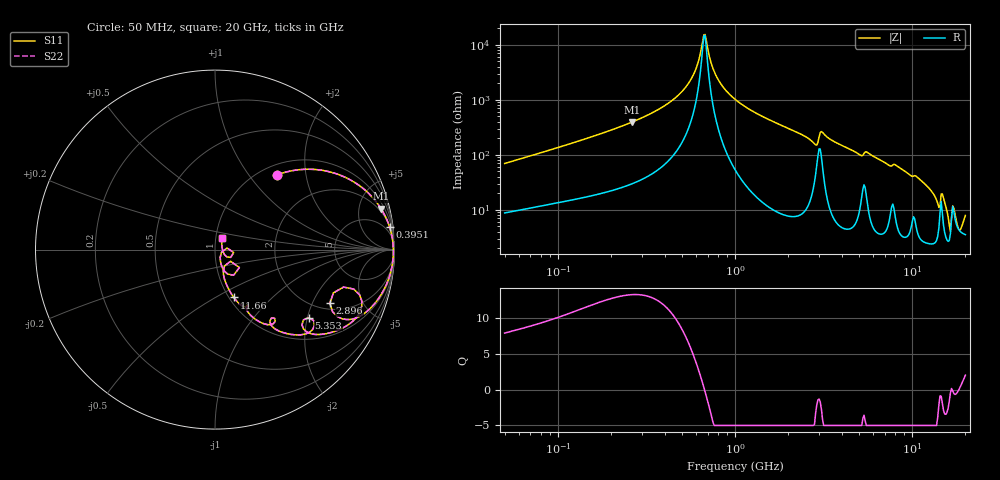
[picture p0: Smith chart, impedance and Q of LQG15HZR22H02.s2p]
!Murata Part Number: LQG15HZR22H02
!These Parameters are Measured in Series Mode Connection
!  o--[Z]--o
!Port1  Port2
!  o-------o
!Freq. Start=50[MHz] Stop=20[GHz], 401[Steps]
# Hz S RI R 50
!Freq.(Hz) S11(Real) S11(Imag) S21(Real) S21(Imag) S12(Real) S12(Imag) S22(Real) S22(Imag)
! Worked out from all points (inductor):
!   401 points, 50 MHz to 20 GHz, reference 50 ohm
!   read as one part in series: L = 215 nH near 51.52 MHz
!   highest Q = 13.2 at 263.7 MHz (marker M1), where L = 240 nH
!   self-resonance near 667.4 MHz
!   S11 on the Smith chart (normalised r, x): 50 MHz: 1.18, +1.38; 395.1 MHz: 2, +15; 2.896 GHz: 2.29, -2.73; 5.353 GHz: 1.57, -2.04; 11.66 GHz: 1.05, -0.61; 20 GHz: 1.07, +0.14
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5e7  0.3448 0.416  0.6552 -0.416  0.6552 -0.416  0.3448 0.416
1.364002e8  0.757 0.3868  0.243 -0.3868  0.243 -0.3868  0.757 0.3868
2.636584e8  0.9254 0.2276  0.0746 -0.2276  0.0746 -0.2276  0.9254 0.2276
3.721004e8  0.9678 0.1405  0.0322 -0.1405  0.0322 -0.1405  0.9678 0.1405
3.95076e8  0.9728 0.1258  0.0272 -0.1258  0.0272 -0.1258  0.9728 0.1258
5.575697e8  0.9907 0.0438  0.00933 -0.0438  0.00933 -0.0438  0.9907 0.0438
6.774326e8  0.9938 -0.00171  0.00619 0.00171  0.00619 0.00171  0.9938 -0.00171
7.868965e8  0.993 -0.037  0.00696 0.037  0.00696 0.037  0.993 -0.037
1e9  0.9857 -0.0954  0.0143 0.0954  0.0143 0.0954  0.9857 -0.0954
2.728004e9  0.7321 -0.3898  0.2679 0.3898  0.2679 0.3898  0.7321 -0.3898
2.896447e9  0.6402 -0.2991  0.3598 0.2991  0.3598 0.2991  0.6402 -0.2991
3.216634e9  0.8136 -0.3333  0.1864 0.3333  0.1864 0.3333  0.8136 -0.3333
4.405649e9  0.6208 -0.4681  0.3792 0.4681  0.3792 0.4681  0.6208 -0.4681
5.352748e9  0.5229 -0.3789  0.4771 0.3789  0.4771 0.3789  0.5229 -0.3789
7.442007e9  0.309 -0.4139  0.691 0.4139  0.691 0.4139  0.309 -0.4139
1.166392e10  0.1048 -0.2668  0.8952 0.2668  0.8952 0.2668  0.1048 -0.2668
1.396067e10  0.0464 -0.1168  0.9536 0.1168  0.9536 0.1168  0.0464 -0.1168
1.504638e10  0.0703 -0.1362  0.9297 0.1362  0.9297 0.1362  0.0703 -0.1362
1.621653e10  0.0289 -0.0434  0.9711 0.0434  0.9711 0.0434  0.0289 -0.0434
1.721783e10  0.0873 -0.0432  0.9127 0.0432  0.9127 0.0432  0.0873 -0.0432
1.855685e10  0.0401 0.00743  0.9599 -0.00743  0.9599 -0.00743  0.0401 0.00743
2e10  0.0386 0.0656  0.9614 -0.0656  0.9614 -0.0656  0.0386 0.0656
